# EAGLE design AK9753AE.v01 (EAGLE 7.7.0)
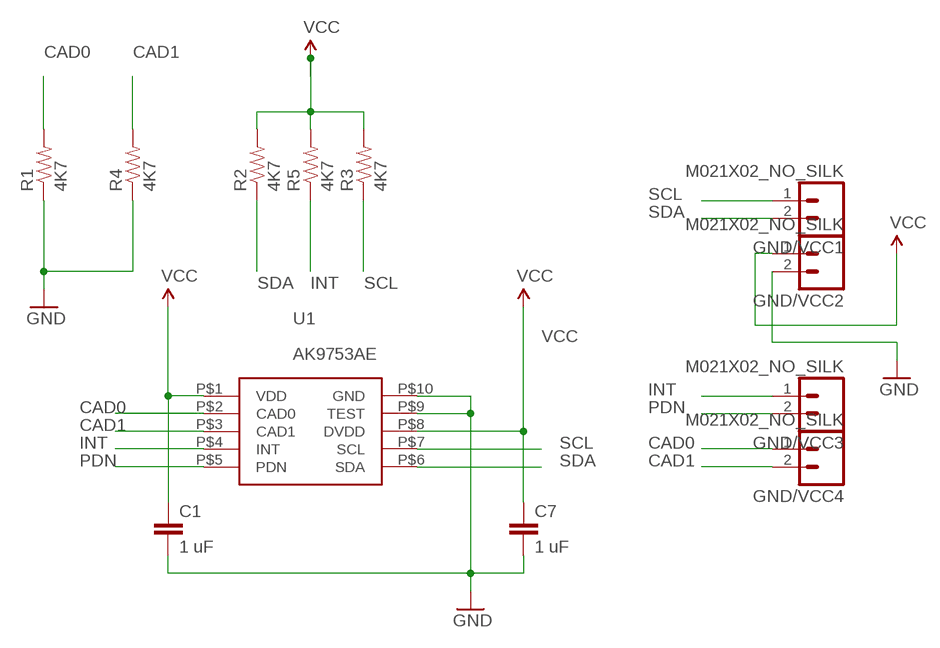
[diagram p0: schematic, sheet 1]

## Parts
C1  1 uF  CAP0402-CAP  [0402-CAP]
C7  1 uF  CAP0402-CAP  [0402-CAP]
GND/VCC1  M021X02_NO_SILK  [1X02_NO_SILK]
GND/VCC2  M021X02_NO_SILK  [1X02_NO_SILK]
GND/VCC3  M021X02_NO_SILK  [1X02_NO_SILK]
GND/VCC4  M021X02_NO_SILK  [1X02_NO_SILK]
R1  4K7  0402RES.KW  [0402-RES]
R2  4K7  0402RES.KW  [0402-RES]
R3  4K7  0402RES.KW  [0402-RES]
R4  4K7  0402RES.KW  [0402-RES]
R5  4K7  0402RES.KW  [0402-RES]
U1  AK9753AE  [AK9753AE]

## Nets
CAD0: GND/VCC4.1 R1.2 U1.P$2(CAD0)
CAD1: GND/VCC4.2 R4.2 U1.P$3(CAD1)
GND: C1.2 C7.2 GND/VCC2.2 R1.1 R4.1 U1.P$9(TEST) U1.P$10(GND)
INT: GND/VCC3.1 R5.1 U1.P$4(INT)
PDN: GND/VCC3.2 U1.P$5(PDN)
SCL: GND/VCC1.1 R3.1 U1.P$7(SCL)
SDA: GND/VCC1.2 R2.1 U1.P$6(SDA)
VCC: C1.1 C7.1 GND/VCC2.1 R2.2 R3.2 R5.2 U1.P$1(VDD) U1.P$8(DVDD)

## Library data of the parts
C1 C7 = SparkFun-Capacitors:CAP: Capacitor
GND/VCC1-GND/VCC4 = SparkFun-Connectors:M02: Standard 2-pin 0.1" header. Use with
R1-R5 = SparkFun-Resistors:0402RES.KW
U1 = kris:AK9753AE: AK9753AE 4x IR Array

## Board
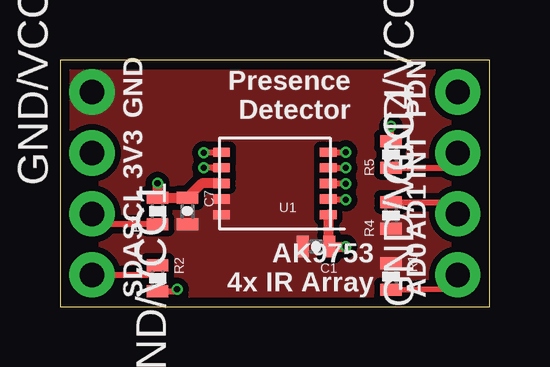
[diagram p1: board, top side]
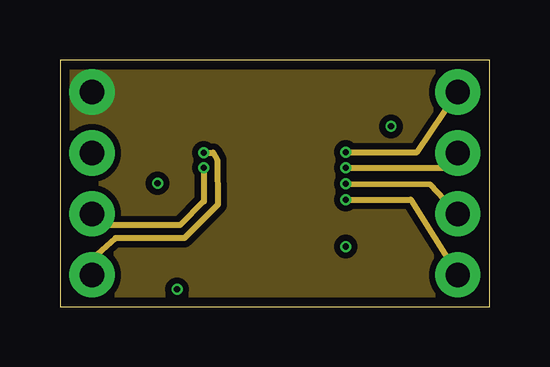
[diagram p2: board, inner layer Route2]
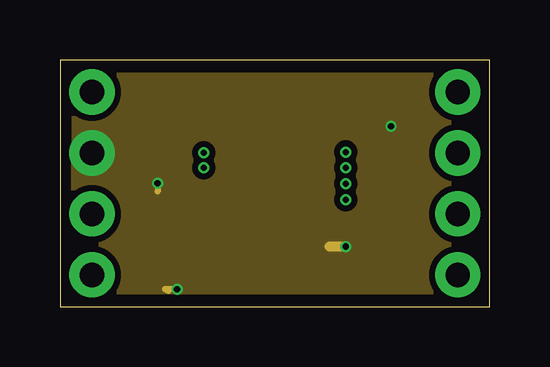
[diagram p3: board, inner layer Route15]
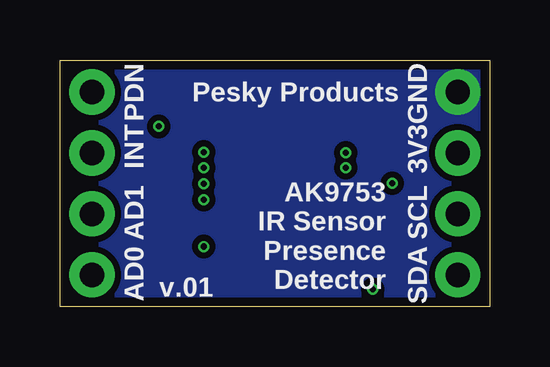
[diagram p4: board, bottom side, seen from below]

Size 17.91 x 10.29 mm. Coordinates in mm from the lower left corner, seen from the top.
Outline: 0,0 17.91,0 17.91,10.29 0,10.29 0,0
Copper layers (1*2*15*16): Top 0.035559375mm / dielectric 0.17018125mm / Route2 0.01778125mm / dielectric 47mil / Route15 0.01778125mm / dielectric 0.17018125mm / Bottom 0.035559375mm
Design rules "OSHPark-4layer *": minimum track width 5mil, minimum drill 10mil, track to track 5mil, track to pad 5mil, pad to pad 5mil, via to via 5mil, smd to smd 5mil, copper to edge 15mil, drill to drill 6mil, minimum pad ring 4mil, minimum via ring 4mil, stop-mask expansion 4mil, vias tented up to drill 20mil, thermal gap 10mil

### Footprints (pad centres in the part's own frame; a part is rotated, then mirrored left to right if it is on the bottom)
0402-CAP = smd 0.5 x 0.9: 1 -0.55,0; 2 0.55,0
1X02_NO_SILK = drill 1.016 pad 1.88: 1 0,0; 2 2.54,0
0402-RES = smd 0.5 x 0.9: 1 -0.55,0; 2 0.55,0
AK9753AE = smd 0.7 x 0.38: P$1 -2.225,1.3; P$2 -2.225,0.65; P$3 -2.225,0; P$4 -2.225,-0.65; P$5 -2.225,-1.3; P$6 2.225,-1.3; P$7 2.225,-0.65; P$8 2.225,0; P$9 2.225,0.65; P$10 2.225,1.3

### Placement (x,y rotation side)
C1  10.67,2.51 180 top
C7  5.31,3.99 270 top
GND/VCC1  1.33,3.87 270 top
GND/VCC2  1.33,6.41 90 top
GND/VCC3  16.57,6.41 90 top
GND/VCC4  16.57,1.33 90 top
R1  13.79,1.27 270 top
R2  4.06,1.19 270 top
R3  4.06,3.99 90 top
R4  13.79,3.81 90 top
R5  13.79,6.35 90 top
U1  8.95,5.14 180 top

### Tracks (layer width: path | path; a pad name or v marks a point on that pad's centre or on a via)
CAD0  (via drill 0.25)
  Top 0.254: 16.54,1.37 GND/VCC4.1 15.94,0.74 R1.2 | U1.P$2 11.81,4.49 v11.91,4.47
  Route2 0.254: v11.91,4.47 14.61,4.47 GND/VCC4.1
CAD1  (via drill 0.25)
  Top 0.254: U1.P$3 11.82,5.14 v11.91,5.13 | R4.2 16.09,4.36 GND/VCC4.2
  Route2 0.254: v11.91,5.13 15.42,5.11 GND/VCC4.2
GND
  pour Bottom (isolate 0.254, no thermals): 0,10.29 17.91,10.29 17.91,0 0.03,0
  pour Route2 (isolate 0.254, no thermals): 0,10.29 17.91,10.29 17.91,0 0.03,0
  pour Top (isolate 0.254, no thermals): 0,10.29 17.91,10.29 17.91,0 0,0
INT  (via drill 0.25)
  Top 0.254: U1.P$4 11.81,5.79 v11.91,5.79 | R5.1 15.96,5.8 GND/VCC3.1
  Route2 0.254: v11.91,5.79 15.95,5.79 GND/VCC3.1
PDN  (via drill 0.25)
  Top 0.254: U1.P$5 v11.9,6.44 v11.91,6.45
  Route2 0.254: v11.91,6.45 14.88,6.45 GND/VCC3.2
SCL  (via drill 0.25)
  Top 0.254: R3.1 1.77,3.44 GND/VCC1.1 | U1.P$7 6.35,5.79 v5.99,5.79
  Route2 0.254: v5.99,5.79 5.99,4.39 5,3.4 1.8,3.4 GND/VCC1.1
SDA  (via drill 0.25)
  Top 0.254: GND/VCC1.2 3.65,1.33 R2.1 | U1.P$6 6.94,6.42 v5.99,6.43
  Route2 0.254: v5.99,6.43 6.38,6.43 6.55,6.14 6.58,4.26 5.18,2.87 2.31,2.87 1.37,2.03 1.37,1.37 GND/VCC1.2
VCC  (via drill 0.25)
  Top 0.254: R2.2 4.81,0.64 v4.88,0.74 | 1.35,6.4 GND/VCC2.1 | 11.71,2.56 v11.91,2.52 | 4.06,5.23 v4.06,5.16 | R5.2 v13.79,7.52 13.79,7.54
  Top 0.406: U1.P$8 5.91,5.14 C7.1 R3.2 v4.06,5.16 | v11.91,2.52 C1.1 11.18,2.81 U1.P$1
  Route15 0.254: v4.88,0.74 4.37,0.74 4.52,0.66 | v4.06,5.16 4.06,4.8 | v13.79,7.52 13.82,7.49 13.79,7.47
  Route15 0.406: v11.91,2.52 C1.1
  pour Route15 (isolate 0.254, no thermals): 0.64,9.65 17.27,9.65 17.2,0.64 0.56,0.64

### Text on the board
tPlace: Presence / Detector | GND | PDN | 3V3 | INT | SCL | AK9753 / 4x IR Array | AD1 | SDA | AD0
bPlace: GND | PDN | Pesky Products | 3V3 | INT | SCL | AK9753 / IR Sensor / Presence / Detector | AD1 | SDA | AD0 | v.01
